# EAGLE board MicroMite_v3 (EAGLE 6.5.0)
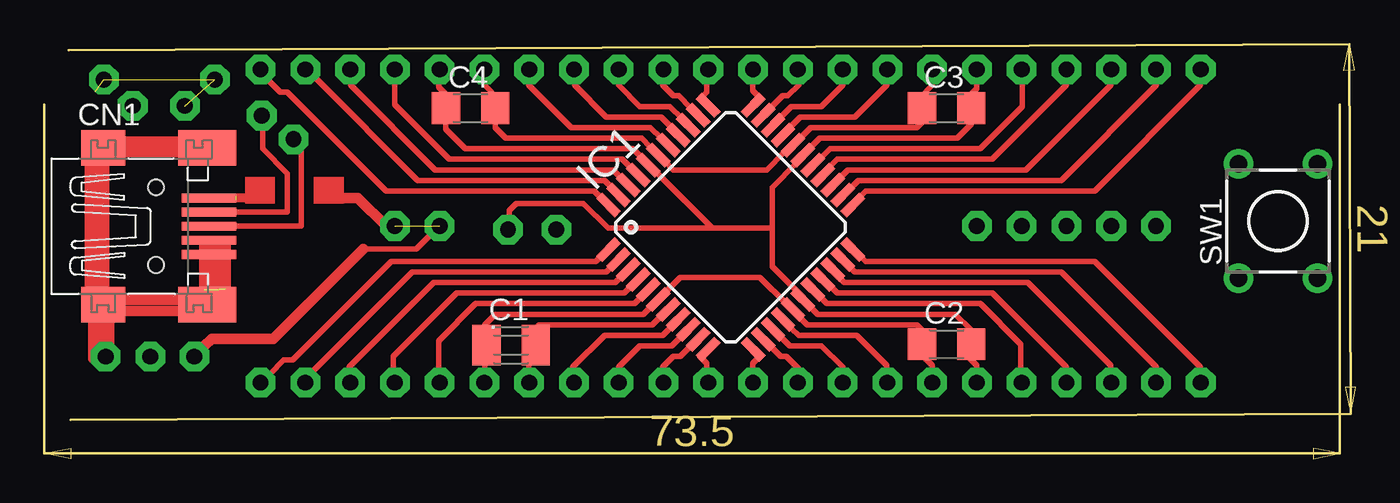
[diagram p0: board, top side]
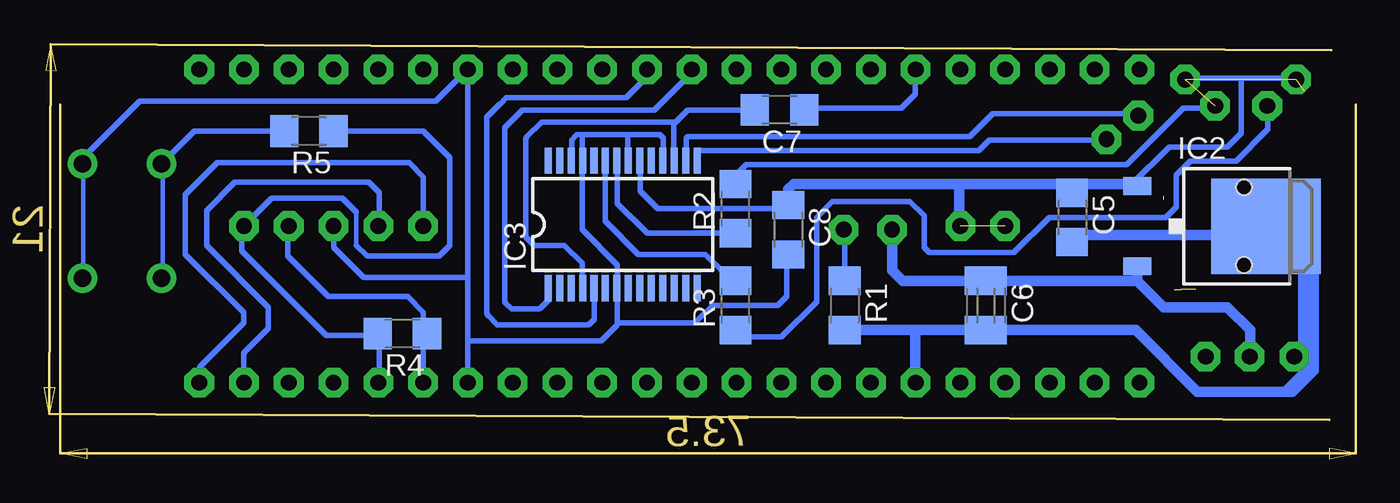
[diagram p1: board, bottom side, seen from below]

Size 74.42 x 23.55 mm. Coordinates in mm from the lower left corner, seen from the top.
Copper layers (1*16): Top 0.035mm / dielectric 1.5mm / Bottom 0.035mm
Design rules "default": minimum track width 10mil, minimum drill 24mil, track to track 8mil, track to pad 8mil, pad to pad 8mil, via to via 8mil, smd to smd 8mil, copper to edge 40mil, drill to drill 8mil, minimum pad ring 10mil, minimum via ring 8mil, stop-mask expansion 4mil, vias tented up to drill 0mil, thermal gap 10mil
Milling: area 0,0 to 1.5,0.6; area 72,0 to 73.5,0.6; area 34,0.7 to 39.5,2.5; area 73.7,22 to 74.3,23.5; area 73.8,2.5 to 74.4,4; area 74.5,11.7 to 76.3,14.4; 6 lines

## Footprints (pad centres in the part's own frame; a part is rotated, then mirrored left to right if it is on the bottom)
C1206 = smd 1.6 x 1.8: 1 -1.4,0; 2 1.4,0
32005-301 = smd 3.1 x 0.5: 1 3,1.6; 2 3,0.8; 3 3,0; 4 3,-0.8; 5 3,-1.6 | smd 2.5 x 2: M1 -3,-4.45; M2 -3,4.45 | smd 3.3 x 2: M3 2.9,4.45; M4 2.9,-4.45 | hole 0.9: 0,2.2; 0,-2.2
TQFP44 = smd 1.5 x 0.5: 1 -5.8,4; 2 -5.8,3.2; 3 -5.8,2.4; 4 -5.8,1.6; 5 -5.8,0.8; 6 -5.8,0; 7 -5.8,-0.8; 8 -5.8,-1.6; 9 -5.8,-2.4; 10 -5.8,-3.2; 11 -5.8,-4; 23 5.8,-4; 24 5.8,-3.2; 25 5.8,-2.4; 26 5.8,-1.6; 27 5.8,-0.8; 28 5.8,0; 29 5.8,0.8; 30 5.8,1.6; 31 5.8,2.4; 32 5.8,3.2; 33 5.8,4 | smd 0.5 x 1.5: 12 -4,-5.8; 13 -3.2,-5.8; 14 -2.4,-5.8; 15 -1.6,-5.8; 16 -0.8,-5.8; 17 0,-5.8; 18 0.8,-5.8; 19 1.6,-5.8; 20 2.4,-5.8; 21 3.2,-5.8; 22 4,-5.8; 34 4,5.8; 35 3.2,5.8; 36 2.4,5.8; 37 1.6,5.8; 38 0.8,5.8; 39 0,5.8; 40 -0.8,5.8; 41 -1.6,5.8; 42 -2.4,5.8; 43 -3.2,5.8; 44 -4,5.8
DPACK_3 = smd 1 x 1.6: 1 -2.28,-4.8; 3 2.28,-4.8 | smd 5.4 x 6.2: 4 0,2.5
SSOP28 = smd 0.4 x 1.5: 1 -4.225,-3.625; 2 -3.575,-3.625; 3 -2.925,-3.625; 4 -2.275,-3.625; 5 -1.625,-3.625; 6 -0.975,-3.625; 7 -0.325,-3.625; 8 0.325,-3.625; 9 0.975,-3.625; 10 1.625,-3.625; 11 2.275,-3.625; 12 2.925,-3.625; 13 3.575,-3.625; 14 4.225,-3.625; 15 4.225,3.625; 16 3.575,3.625; 17 2.925,3.625; 18 2.275,3.625; 19 1.625,3.625; 20 0.975,3.625; 21 0.325,3.625; 22 -0.325,3.625; 23 -0.975,3.625; 24 -1.625,3.625; 25 -2.275,3.625; 26 -2.925,3.625; 27 -3.575,3.625; 28 -4.225,3.625
TL1105 = drill 1 pad 1.676: 1 -2.25,3.25; 2 2.25,3.25; 3 -2.25,-3.25; 4 2.25,-3.25

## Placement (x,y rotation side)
.  [C1206]  26.5,6.2 0 top
..  [C1206]  21.3,8.7 270 bottom
C1  47uF  [C1206]  26.5,6.7 0 top
C2  100nF  [C1206]  51.2,6.5 0 top
C3  100nF  [C1206]  51.2,19.9 0 top
C4  100nF  [C1206]  24.2,19.9 0 top
C5  100nF  [C1206]  16.1,13.7 270 bottom
C6  47uF  [C1206]  20.7,8.7 270 bottom
C7  110nF  [C1206]  32.7,19.8 180 bottom
C8  100nF  [C1206]  32.2,13 270 bottom
CN1  USB  [32005-301]  6.36,13.2 0 top
IC1  PIC32MX150D  [TQFP44]  38.95,13.14 45 top
IC2  LF33  [DPACK_3]  7.6,13.2 270 bottom
IC3  FT232RL  [SSOP28]  41.6,13.3 0 bottom
R1  330R  [C1206]  29,8.7 270 bottom
R2  330R  [C1206]  35.2,14.2 90 bottom
R3  330R  [C1206]  35.2,8.7 90 bottom
R4  10K  [C1206]  54.1,7.1 180 bottom
R5  100R  [C1206]  59.4,18.6 180 bottom
SW1  [TL1105]  70,13.5 0 top

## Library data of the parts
. .. C1-C8 R1-R5 = resistor
CN1 = con-cypressindustries
IC1 = microchip
IC2 = linear
IC3 = analog-devices
SW1 = switch

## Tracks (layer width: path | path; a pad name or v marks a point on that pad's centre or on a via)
PIN1  (via drill 0.9 pad 1.68)
  other vias: 63.08,13.21
S$1
  Top 0.305: 65.6,21.5 65.6,21.2 59.6,15.2 46.6,15.2 45.6,14.2
S$2
  Top 0.305: 58,21.5 58,21.2 53.8,17 45,17 44,16
S$3
  Top 0.305: 65.6,5 65.6,5.2 59.6,11.2 46.6,11.2 46.2,11.6
S$4
  Top 0.305: 45.2,14.8 46.2,15.8 57.7,15.8 63.1,21.2 63.1,21.4
S$5
  Top 0.305: 45.3,21.4 45.3,21.2 44.1,20 42.4,20 41.2,18.8
S$6
  Top 0.305: 42.9,8 43.3,7.6 49.5,7.6 49.9,7.2
S$7  (via drill 0.9 pad 1.68)
  other vias: 40.22,4.32
S$8
  Top 0.305: 45.6,11 46,10.6 57.7,10.6 63.1,5.2 63.1,5
S$9
  Top 0.305: 45,10.4 45.4,10 55.8,10 60.5,5.3 60.5,5
S$10
  Top 0.305: 58,5 58,5.2 53.8,9.4 45,9.4 44.6,9.8
S$11
  Top 0.305: 44,9.2 44.4,8.8 53.1,8.8 55.4,6.5 55.4,5
S$12
  Top 0.305: 42.4,7.4 42.8,7 46.1,7 47.8,5.3 47.8,5
S$13
  Top 0.305: 42.4,6.4 44.1,6.4 45.3,5.2 45.3,5.1
S$14
  Top 0.305: 42.8,5 42.8,5.1 42.1,5.8 41.8,5.8 41.2,6.4
S$15  (via drill 0.9 pad 1.68)
  other vias: 47.84,4.32
S$16
  Top 0.305: 42.9,18.2 43.5,18.8 49.5,18.8 49.9,19.2
S$17
  Top 0.305: 43.4,16.4 44.6,17.6 53.1,17.6 55.5,20 55.5,21.5
S$18
  Top 0.305: 42.8,17 44,18.2 51.8,18.2 52.6,19 52.6,19.2 52.5,19.3
S$19
  Top 0.305: 41.2,19.9 41.9,20.6 42.2,20.6 42.8,21.2 42.8,21.4
S$21
  Top 0.305: 42.3,18.8 42.9,19.4 46,19.4 47.8,21.2 47.8,21.4
S$22
  Top 0.305: 60.5,21.4 60.5,21.2 55.7,16.4 45.6,16.4 44.6,15.4
S$23
  Top 0.305: 40.6,20.5 40.2,20.9 40.2,21.5
S$24
  Top 0.305: 37.3,20.5 37.6,20.8 37.6,21.4
S$25
  Top 0.305: 35.1,21.3 35.1,21.2 35.7,20.6 36,20.6 36.7,19.9
S$26
  Top 0.305: 32.6,21.3 32.6,21.2 33.8,20 35.5,20 36.2,19.3
S$27
  Top 0.305: 30.1,21.3 30.1,21.2 31.9,19.4 35,19.4 35.6,18.8
S$28  (via drill 0.9 pad 1.68)
  other vias: 42.76,22.1
S$29
  Top 0.305: 27.5,21.4 27.5,21.2 29.9,18.8 34.4,18.8 35,18.2
S$30
  Top 0.305: 34.4,17.7 33.9,18.2 26.2,18.2 25.6,18.8 25.6,19.3
S$31
  Top 0.305: 25,21.4 25,21.2 25.8,20.4
S$32
  Top 0.305: 33.3,16.5 32.8,17 23,17 19.9,20.1 19.9,21.4
S$33
  Top 0.305: 17.4,21.3 17.4,21.2 22.2,16.4 32.3,16.4 32.7,16
S$34
  Top 0.305: 32.2,15.4 31.8,15.8 21.2,15.8 15.4,21.6
S$35
  Bottom 0.305: 43.9,10.3 43.9,11.1 44.9,12.1 46.6,12.1 47.1,12.6 47.1,18.09 arc45 47.03,18.27 46.2,19.1 38.6,19.1 | 38.7,17.5 38.7,19 38.6,19.1 | 38.6,19.1 37.9,19.8 34.7,19.8
S$36
  Top 0.305: 33.9,9.2 33.5,8.8 24.5,8.8 22.4,6.7 22.4,5
S$37
  Top 0.305: 34.5,8.7 34,8.2 25.6,8.2 25,7.6 25,5
S$38  (via drill 0.9 pad 1.68)
  other vias: 45.3,22.1
S$39  (via drill 0.9 pad 1.68)
  other vias: 47.84,22.1
S$40  (via drill 0.9 pad 1.68)
  other vias: 50.38,22.1
S$41  (via drill 0.9 pad 1.68)
  other vias: 52.92,22.1
S$42  (via drill 0.9 pad 1.68)
  other vias: 55.46,22.1
S$43  (via drill 0.9 pad 1.68)
  other vias: 58,22.1
S$44  (via drill 0.9 pad 1.68)
  other vias: 60.54,22.1
S$45  (via drill 0.9 pad 1.68)
  other vias: 63.08,22.1
S$46  (via drill 0.9 pad 1.68)
  other vias: 65.62,22.1
S$47  (via drill 0.9 pad 1.68)
  other vias: 40.22,22.1
S$48  (via drill 0.9 pad 1.68)
  other vias: 37.68,22.1
S$49  (via drill 0.9 pad 1.68)
  other vias: 35.14,22.1
S$50  (via drill 0.9 pad 1.68)
  other vias: 32.6,22.1
S$51  (via drill 0.9 pad 1.68)
  other vias: 30.06,22.1
S$52  (via drill 0.9 pad 1.68)
  other vias: 27.52,22.1
S$53  (via drill 0.9 pad 1.68)
  other vias: 24.98,22.1
S$54  (via drill 0.9 pad 1.68)
  other vias: 22.44,22.1
S$55  (via drill 0.9 pad 1.68)
  other vias: 19.9,22.1
S$56  (via drill 0.9 pad 1.68)
  other vias: 17.36,22.1
S$57  (via drill 0.9 pad 1.68)
  other vias: 14.82,22.1
S$58  (via drill 0.9 pad 1.68)
  other vias: 12.28,22.1
S$59  (via drill 0.9 pad 1.68)
  other vias: 37.68,4.32
S$60  (via drill 0.9 pad 1.68)
  other vias: 35.14,4.32
S$61  (via drill 0.9 pad 1.68)
  other vias: 32.6,4.32
S$62  (via drill 0.9 pad 1.68)
  other vias: 30.06,4.32
S$63  (via drill 0.9 pad 1.68)
  other vias: 27.52,4.32
S$64  (via drill 0.9 pad 1.68)
  other vias: 24.98,4.32
S$65  (via drill 0.9 pad 1.68)
  other vias: 22.44,4.32
S$66  (via drill 0.9 pad 1.68)
  other vias: 19.9,4.32
S$67  (via drill 0.9 pad 1.68)
  other vias: 17.36,4.32
S$68  (via drill 0.9 pad 1.68)
  other vias: 14.82,4.32
S$69  (via drill 0.9 pad 1.68)
  other vias: 12.28,4.32
S$70  (via drill 0.9 pad 1.68)
  other vias: 42.76,4.32
S$71  (via drill 0.9 pad 1.68)
  other vias: 45.3,4.32
S$72  (via drill 0.9 pad 1.68)
  other vias: 50.38,4.32
S$73  (via drill 0.9 pad 1.68)
  other vias: 52.92,4.32
S$74  (via drill 0.9 pad 1.68)
  other vias: 55.46,4.32
S$75  (via drill 0.9 pad 1.68)
  other vias: 58,4.32
S$76  (via drill 0.9 pad 1.68)
  other vias: 60.54,4.32
S$77  (via drill 0.9 pad 1.68)
  other vias: 63.08,4.32
S$78  (via drill 0.9 pad 1.68)
  other vias: 65.62,4.32
S$79
  Top 0.305: 42.3,6.4 41.7,7
S$80
  Bottom 0.61: 15.4,12.7 7.7,12.7
S$81  (via drill 0.9 pad 1.68)
  other vias: 60.54,13.21
S$82  (via drill 0.9 pad 1.68)
  other vias: 58,13.21
S$83  (via drill 0.9 pad 1.68)
  other vias: 55.46,13.21
S$84  (via drill 0.9 pad 1.68)
  other vias: 52.92,13.21
S$85
  Top 0.305: 18.1,11.9 21.1,11.9 21.9,12.7
  Top 0.61: 18.1,11.9 13,6.8 9.5,6.8 9.1,6.4
S$86
  Bottom 0.305: 50.8,21.6 50.9,21.6 52.2,20.3 69,20.3 72.1,17.2
S$87
  Top 0.305: 50.4,21.4 50.4,21.2 49.7,20.5
S$88
  Top 0.305: 40.6,5.8 40.2,5.4 40.2,5
S$89
  Top 0.305: 37.2,5.8 37.6,5.4 37.6,5
S$90
  Top 0.305: 35,8.1 34.5,7.6 28.1,7.6 27.5,7 27.5,5.1
S$91
  Top 0.305: 32.6,4.9 32.6,5.2 33.8,6.4 35.6,6.4 36.2,7
S$92
  Top 0.305: 30,5 30,5.2 31.8,7 35.1,7 35.6,7.5
S$93
  Bottom 0.61: 3,8.5 3,6.4
S$94
  Top 0.305: 32.2,10.9 31.9,10.6 20.9,10.6 15.3,5
S$95
  Top 0.305: 50.4,5 50.4,5.3 49.6,6.1
S$96
  Top 0.305: 52.6,7.3 51.7,8.2 43.9,8.2 43.5,8.6
S$97
  Top 0.305: 52.9,5.1 52.9,5.3 52.5,5.7
S$98
  Top 0.305: 52.9,21.4 52.9,21 52.6,20.7
S$99
  Top 0.305: 17.3,5.1 17.3,5.2 22.1,10 32.4,10 32.8,10.4
S$100
  Top 0.305: 35.1,5 35.1,5.2 35.7,5.8 36.1,5.8 36.7,6.4
S$101
  Top 0.305: 10.8,13.2 14.6,13.2 14.6,17.6
S$102
  Bottom 0.305: 63.1,5.1 63.1,6 61.7,7.4 61.7,8.6 65.2,12.1 65.2,14.1 63.6,15.7 56,15.7 55.4,15.1 55.4,13.9
S$103
  Bottom 0.61: 3,8.6 3,10.8 3.2,11 3,11 2.8,10.8 2.8,8.4 2.6,8.2
S$104
  Bottom 0.305: 52.9,14 52.9,16 53.7,16.8 64.6,16.8 66.4,15 66.4,11.6 63.1,8.3 63.1,7.7 65.6,5.2 65.6,4.9
S$105
  Bottom 0.305: 67.2,17.2 67.2,17.3 65.9,18.6 60.8,18.6 60.7,18.7
S$106
  Bottom 0.305: 63.2,12.6 63.2,11.8 58.4,7 55.7,7 55.6,6.9
S$107
  Top 0.305: 42,17.4 41,16.4 35.7,16.4 35.2,16.9
S$108
  Top 0.305: 22.4,21.4 22.4,21.1 22.8,20.7
S$109
  Top 0.305: 42.1,8.8 40.6,10.3 36.1,10.3 35.3,9.5
S$110
  Top 0.305: 22.8,19.1 22.8,18.7 23.9,17.6 26,17.6 26.3,17.6 33.4,17.6 33.9,17.1
S$111
  Bottom 0.305: 13.1,19.6 20.6,19.6 21.9,18.3 37.9,18.3 38,18.2 38,17.4
S$112
  Bottom 0.305: 34.8,6.9 32.6,6.9 30.6,8.9 30.6,13.7 29.7,14.6 25.3,14.6 24.5,13.8 24.5,12 24.2,11.7 19.4,11.7 17.4,13.7 10.8,13.7 10.2,14.3 10.2,16.1 9.4,16.9 6.8,16.9 5,18.7 5,19.2
S$113  (via drill 0.9 pad 1.68)  (1 unrouted)
  other vias: 22.44,13.21 19.9,13.21
S$114  (via drill 0.9 pad 1.68)
  other vias: 12.35,19.48
S$115  (via drill 0.9 pad 1.68)
  other vias: 26.32,13.01
S$116  (via drill 0.9 pad 1.68)
  other vias: 29.06,13.01
S$117  (via drill 0.9 pad 1.68)
  other vias: 14.15,18.14
S$118  (via drill 0.9 pad 1.68)
  other vias: 5.03,20.03
S$119  (via drill 0.9 pad 1.68)
  other vias: 3.49,5.79
S$120
  Bottom 0.305: 57.8,18.6 52.9,18.6 51.4,17.1 51.4,12.1 52,11.5 56.1,11.5 56.7,12.1
S$121  (via drill 0.9 pad 1.68)
  other vias: 6.03,5.79 8.53,5.79
S$122  (via drill 0.9 pad 1.68)  (3 unrouted)
  other vias: 7.99,20.03 3.39,21.53 9.69,21.53
S$123
  Bottom 0.305: 13.3,16.7 34.6,16.7 35.3,16 35.3,15.2
S$124
  Bottom 0.305: 29,10.5 28.9,10.4
S$125
  Top 0.305: 31.6,14.8 31.2,15.2 19.4,15.2 13.8,20.8 13.4,20.8 12.6,21.6
S$126
  Top 0.61: 16,14.8 17.8,14.8 19.4,13.2
S$127
  Top 0.305: 10.7,14 13.8,14 13.8,16.2 12.4,17.6 12.4,18.8
S$128
  Bottom 0.305: 45.8,9 46.23,8.57 arc45 46.41,8.5 47.9,8.5 48.23,8.83 arc45 48.3,9 48.3,18.8 47.3,19.8 39.8,19.8 38.1,21.5
S$129
  Bottom 0.305: 37.3,17.5 21.4,17.5 20.8,18.1 14.9,18.1
S$130
  Bottom 0.305: 32.2,14.9 32.2,15.3 32.2,15.4
  Bottom 0.61: 31.9,15.6 32.2,15.3 32.2,14.8
S$131
  Bottom 0.305: 9,3.8 3.8,3.8 2.4,5.2 2.4,10.6
  Bottom 0.61: 25,7.3 25,5.1 | 25,7.3 12.5,7.3 9,3.8 3.6,3.8 2.4,5 2.4,5.2 2.4,10.8 | 25,7.3 28.7,7.3
S$132
  Bottom 0.305: 41.9,7.7 37.5,7.7 36.5,8.7 32.8,8.7 32.3,9.2
S$133
  Bottom 0.305: 58,12.6 58,12 56.3,10.3 50.4,10.3 | 50.4,4.8 50.4,10.3 | 50.4,10.3 50.4,21.5
S$134
  Bottom 0.61: 22.5,13.9 22.5,15.5
S$135  (1 unrouted)
  Top 0.305: 10.9,14.9 11.7,14.9 | 10.9,14.7 11.7,14.7
S$136
  Top 0.305: 34.7,16.3 37.9,13.1 | 37.9,13.1 32,13.1 30.6,14.5 26.8,14.5 26.4,14.1 26.4,13.7 | 42.7,16.8 41.3,15.4 41.3,13.1 | 42.8,9.4 41.3,10.9 41.3,13.1 | 37.9,13.1 41.3,13.1
S$137
  Top 0.305: 31.6,11.5 31.3,11.2 19.7,11.2 14.1,5.6 13.6,5.6 12.8,4.8
S$138
  Bottom 0.305: 32.3,10.8 32.3,9.3
S$140
  Bottom 0.61: 2.8,8.1 2.8,5 3.9,3.9
S$142
  Bottom 0.305: 35.9,10.6 36.9,11.6 40.7,11.6 42.6,13.5 42.6,16.3
S$143
  Top 0.305: 9.4,17.4 8.8,17.4 8.6,17.6 8.2,17.6 3.4,17.6
  Top 0.61: 4.8,17.8 8,17.8 8.2,17.6 8,17.4 4.6,17.4
S$144
  Bottom 0.305: 12.4,10.8 12.2,11
  Bottom 0.61: 20.1,10.1 12.4,10.1 | 6,6.4 6,7.3 7.3,8.6 10.9,8.6 12.4,10.1 | 12.4,10.8 12.4,10.1
S$145
  Bottom 0.61: 13,15.6 31.8,15.6
S$146
  Bottom 0.305: 12.2,15.4 12,15.2
S$147
  Top 0.305: 19.8,5 19.8,5.8 23.4,9.4 32.9,9.4 33.3,9.8
S$148
  Bottom 0.305: 29,12.2 29,10.1
S$149
  Top 0.61: 3,17 3,9.4 3.8,9.4
S$150
  Top 0.61: 4.4,18 8.4,18
S$151  (3 unrouted)
  Top 0.61: 9.1,9.6 9.1,12.2 | 9.5,9.6 9.5,12.2 | 9.9,9.6 9.9,12.2 | 10.3,9.6 10.3,12.2
S$152
  Bottom 0.305: 13.3,16.7 13,16.7 9.8,19.9 8.5,19.9
S$153
  Bottom 0.305: 4.1,21.6 6.5,21.6 | 6.5,21.6 8.9,21.6 | 6.5,21.6 6.5,18.5 7.3,17.7 10.6,17.7 12.8,15.5
S$154
  Bottom 0.61: 22,10.1 25.7,10.1 26.3,10.7 26.3,12.2
S$155
  Top 0.61: 2.6,16.8 2.6,9.4
S$156
  Top 0.61: 3.4,16.6 3.4,9.8
S$157
  Top 0.305: 9.6,8.6 9.4,8.8 8.2,8.8
  Top 0.61: 4.2,9 8,9 8.2,8.8 8.2,8.6 8,8.4 4.4,8.4 4.2,8.6
S$158
  Top 0.61: 3.7,8.1 3.7,7.4 | 3.7,6.5 3.7,7.4 | 3.7,7.4 3.2,7.9 3.2,7.4 | 3.2,6.5 3.2,7.4 | 3.2,7.4 2.8,7.8 2.8,5.7
S$159
  Bottom 0.305: 41.9,16.2 41.9,14.5 40.2,12.8 35.9,12.8
S$161
  Bottom 0.305: 48.5,20.2 48.2,20.5 41.4,20.5 40.5,21.4
S$162
  Bottom 0.305: 48.57,20.13 49.3,19.4 49.3,8.3 arc-45 49.23,8.13 48.7,7.6 43.61,7.6 arc-45 43.43,7.67 43.2,7.9 43.2,9
S$163
  Bottom 0.305: 41.9,8.9 41.9,7.7 arc45 41.97,7.53 42.8,6.7 50.3,6.7
S$166
  Bottom 0.305: 41.3,17.6 41.3,18.4 | 39.3,17.6 39.3,18.2 39.5,18.4 41.3,18.4 | 44.5,17.6 44.5,18.1 44.2,18.4 43.9,18.4 | 41.3,18.4 43.9,18.4 | 43.9,17.6 43.9,18.4
S$168
  Bottom 0.305: 55.4,5 55.4,7.1
S$170
  Bottom 0.254: 56.7,14 56.7,12.2
  Bottom 0.305: 62.6,13.7 61.5,14.8 57.5,14.8 56.7,14
S$171
  Bottom 0.305: 31.4,19.9 25.8,19.9 25,20.7 25,21.4
S$172
  Bottom 0.305: 8,13.4 8,13.1
S$173
  Bottom 0.305: 52.9,5.1 52.9,8.3 53.8,9.2 53.9,9.2 54.1,9.2 58.3,9.2 60.6,11.5 60.6,12.5
S$174
  Bottom 0.305: 40.6,16.3 40.6,15.2 39.6,14.2 32.9,14.2
S$175
  Bottom 0.254: 67.7,16.1 67.7,10.9
S$176
  Bottom 0.305: 43.9,16.3 43.9,13 41.9,11 41.9,10.2
S$177
  Bottom 0.254: 72.2,16.1 72.2,10.9
(copper drawn outside any net)
  shapes: Top area x2

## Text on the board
tFinish: > | < | 44 | 43 | 42 | 41 | 40 | 39 | 38 | 37 | 36 | 35 | 34 | 33 | 32 | 31 | 30 | 29 | 28 | 27 | 26 | 25 | 24 | 23 | ^ | Reset | 0v | 3.3 | 5v | OUTPUT | 1 | 2 | 3 | 4 | 5 | 6 | 7 | 8 | 9 | 10 | 11 | 12 | 13 | 14 | 15 | 16 | 17 | 18 | 19 | 20 | 21 | 22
